(* Logix 5000 AddOnInstructionDefinition export Banner_IOLM_Param_C_v5; software revision 33.00 *)

TYPE Banner_IOL_Port_v5 :   // UDT that has all of the data items necessary to communicate with a specific Port on a IO-Link Master
STRUCT
   Port_Controlled : INT;   // Each bit represents a port on an IO-Link Master. Set to 1 to tell AOI to control that port.
   Port_Activate : INT;   // Each bit represents a port on an IO-Link Master. When ON that port will process any commands in queue.
   Port_Read : INT;   // Each bit represents a port on an IO-Link Master. Used to determine when device AOI has requested a Read command.
   Port_Write : INT;   // Each bit represents a port on an IO-Link Master. Used to determine when device AOI has requested a Write command.
   Port_RW_Complete : INT;   // Each bit represents a port on an IO-Link Master. Tells device AOI that Read or Write request has been completed.
   Port_Device_Read : INT;
   Data_Transfer : SINT[250];   // Array to transfer data from IO-Master to device AOIs.
END_STRUCT
END_TYPE

TYPE Banner_IOLM_EL_v5 :   // Error Log for Messages to IOLM.
STRUCT
   RW : SINT;   // 0 = Read, 1 = Write.
   Port : SINT;   // Port number that generated error.
   Index : INT;   // IO-Link Index for generated error.
END_STRUCT
END_TYPE

TYPE Banner_IOLMC_v5 :   // UDT to control IO-Link Masters. Modified for Comtrol Masters.
STRUCT
   Message_Source_Data : SINT[520];   // Array used to generate the source data for an Explicit Message
   Message_Destination_Data : SINT[520];   // Array that stores the data from the IO-Link sensor for an Explicit Message.
   Error_Log : Banner_IOLM_EL_v5[10];
   Error_Write_Retry : BOOL;
   Num_Error_MSGS : DINT;   // 0 = While waiting for a command, 1 = Processing command
   IO_Link_Master_Busy : BOOL;
   AOI_Reset : BOOL;   // Resets AOI.
   Port_Data : Banner_IOL_Port_v5;
   Halt_Operation : BOOL;
   AOI_Halted : BOOL;
END_STRUCT
END_TYPE

ADD_ON_INSTRUCTION Banner_IOLM_Param_C_v5   (* revision 5.0, vendor Banner Engineering *)
// AOI that controls a Comtrol IO-Link Master with Banner devices for parameter data operations.
VAR_IN_OUT
   Message : MESSAGE; {required}   // Message used to gather data from a device plugged into an Allen Bradley IO-Link Master.
   IOLM : Banner_IOLMC_v5; {required}
END_VAR
VAR_INPUT
   Port1 : BOOL; {required}
   Port2 : BOOL; {required}
   Port3 : BOOL; {required}
   Port4 : BOOL; {required}
   Port5 : BOOL; {required}
   Port6 : BOOL; {required}
   Port7 : BOOL; {required}
   Port8 : BOOL; {required}
END_VAR
VAR_OUTPUT
   Done : BOOL; {visible}
   Busy : BOOL; {visible}
   Error : BOOL; {visible}
END_VAR
VAR
   Lock : DINT; {access None}
   Disable_Timer : BOOL; {access None}
   Byte_Length : SINT; {access None}
   Current_Port : INT; {access None}   // Current port to communicate with via the IO-Link Master.
   Array_Index : DINT; {access None}
   Data_Index : DINT; {access None}
   Message_Timer : TIMER := (PRE := 100); {access None}
   Message_Timer2 : TIMER := (PRE := 5000); {access None}
   Error_Index : DINT; {access None}
   Temp_Index : INT; {access None}
   Timer8 : TIMER := (PRE := 3000); {access None}
   WriteCnt : DINT; {access None}
   Last_Index : DINT; {access None}
   WrCntTotal : DINT; {access None}
END_VAR

ROUTINE Logic   (* ladder *)
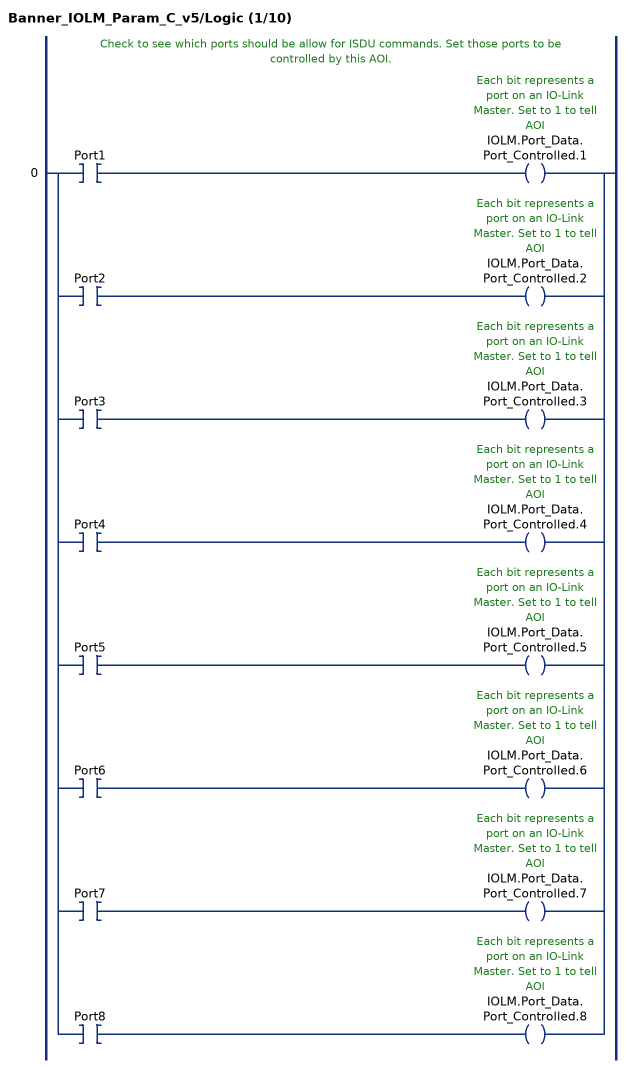
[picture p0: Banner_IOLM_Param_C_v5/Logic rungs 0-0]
   // Check to see which ports should be allow for ISDU commands. Set those ports to be controlled by this AOI.
   0: [XIC(Port1) OTE(IOLM.Port_Data.Port_Controlled.1) ,XIC(Port2) OTE(IOLM.Port_Data.Port_Controlled.2) ,XIC(Port3) OTE(IOLM.Port_Data.Port_Controlled.3) ,XIC(Port4) OTE(IOLM.Port_Data.Port_Controlled.4) ,XIC(Port5) OTE(IOLM.Port_Data.Port_Controlled.5) ,XIC(Port6) OTE(IOLM.Port_Data.Port_Controlled.6) ,XIC(Port7) OTE(IOLM.Port_Data.Port_Controlled.7) ,XIC(Port8) OTE(IOLM.Port_Data.Port_Controlled.8) ];
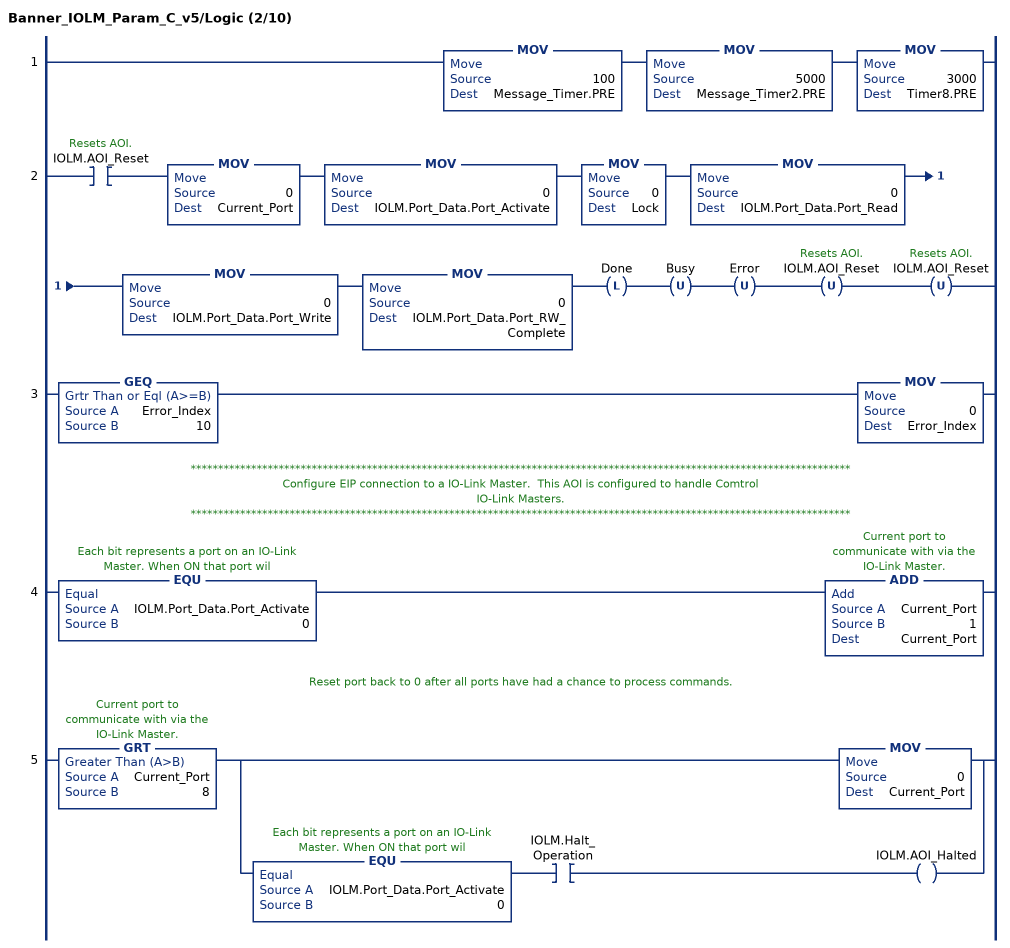
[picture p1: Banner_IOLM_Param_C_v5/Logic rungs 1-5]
   1: MOV(100,Message_Timer.PRE)MOV(5000,Message_Timer2.PRE)MOV(3000,Timer8.PRE);
   2: XIC(IOLM.AOI_Reset)MOV(0,Current_Port)MOV(0,IOLM.Port_Data.Port_Activate)MOV(0,Lock)MOV(0,IOLM.Port_Data.Port_Read)MOV(0,IOLM.Port_Data.Port_Write)MOV(0,IOLM.Port_Data.Port_RW_Complete)OTL(Done)OTU(Busy)OTU(Error)OTU(IOLM.AOI_Reset)OTU(IOLM.AOI_Reset);
   3: GEQ(Error_Index,10)MOV(0,Error_Index);
   // ************************************************************************************************************************
   // Configure EIP connection to a IO-Link Master.  This AOI is configured to handle Comtrol
   // IO-Link Masters.
   // ************************************************************************************************************************
   4: EQU(IOLM.Port_Data.Port_Activate,0)ADD(Current_Port,1,Current_Port);
   // Reset port back to 0 after all ports have had a chance to process commands.
   5: GRT(Current_Port,8)[MOV(0,Current_Port) ,EQU(IOLM.Port_Data.Port_Activate,0) XIC(IOLM.Halt_Operation) OTE(IOLM.AOI_Halted) ];
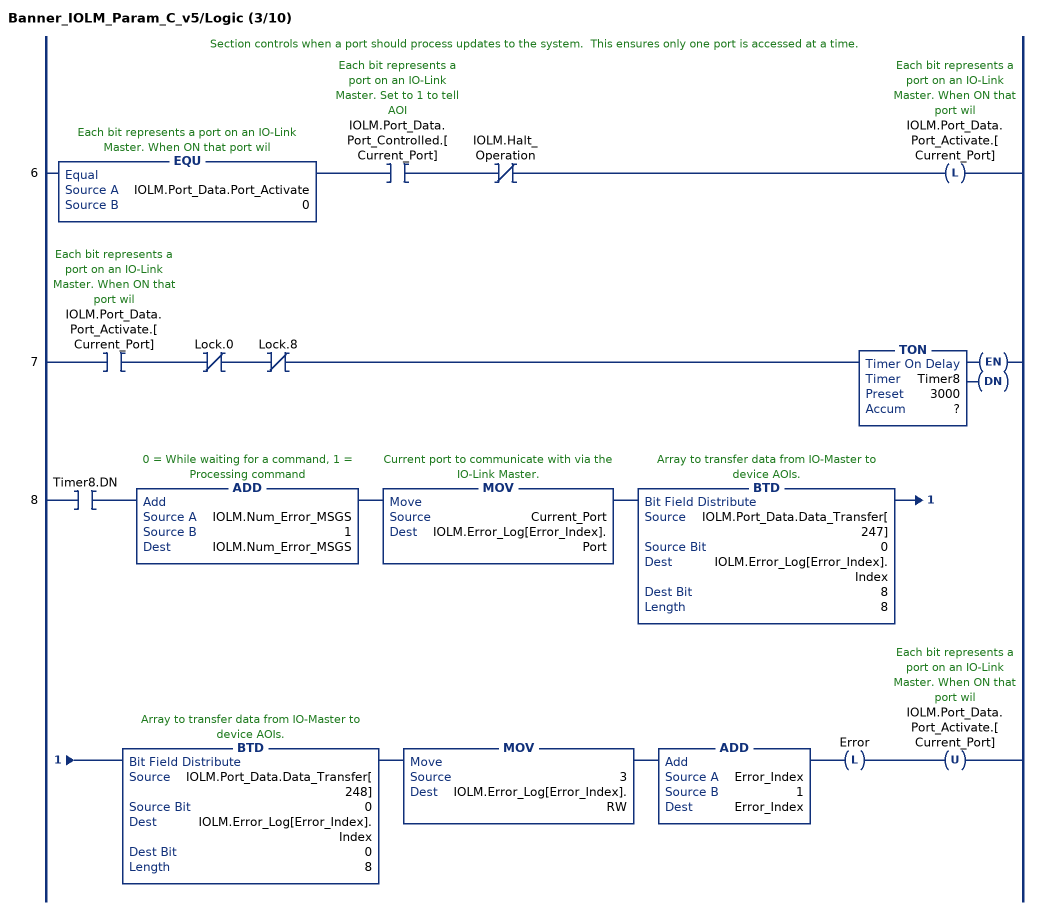
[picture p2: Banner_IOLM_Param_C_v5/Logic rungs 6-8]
   // Section controls when a port should process updates to the system.  This ensures only one port is accessed at a time.
   6: EQU(IOLM.Port_Data.Port_Activate,0)XIC(IOLM.Port_Data.Port_Controlled.[Current_Port])XIO(IOLM.Halt_Operation)OTL(IOLM.Port_Data.Port_Activate.[Current_Port]);
   7: XIC(IOLM.Port_Data.Port_Activate.[Current_Port])XIO(Lock.0)XIO(Lock.8)TON(Timer8,?,?);
   8: XIC(Timer8.DN)ADD(IOLM.Num_Error_MSGS,1,IOLM.Num_Error_MSGS)MOV(Current_Port,IOLM.Error_Log[Error_Index].Port)BTD(IOLM.Port_Data.Data_Transfer[247],0,IOLM.Error_Log[Error_Index].Index,8,8)BTD(IOLM.Port_Data.Data_Transfer[248],0,IOLM.Error_Log[Error_Index].Index,0,8)MOV(3,IOLM.Error_Log[Error_Index].RW)ADD(Error_Index,1,Error_Index)OTL(Error)OTU(IOLM.Port_Data.Port_Activate.[Current_Port]);
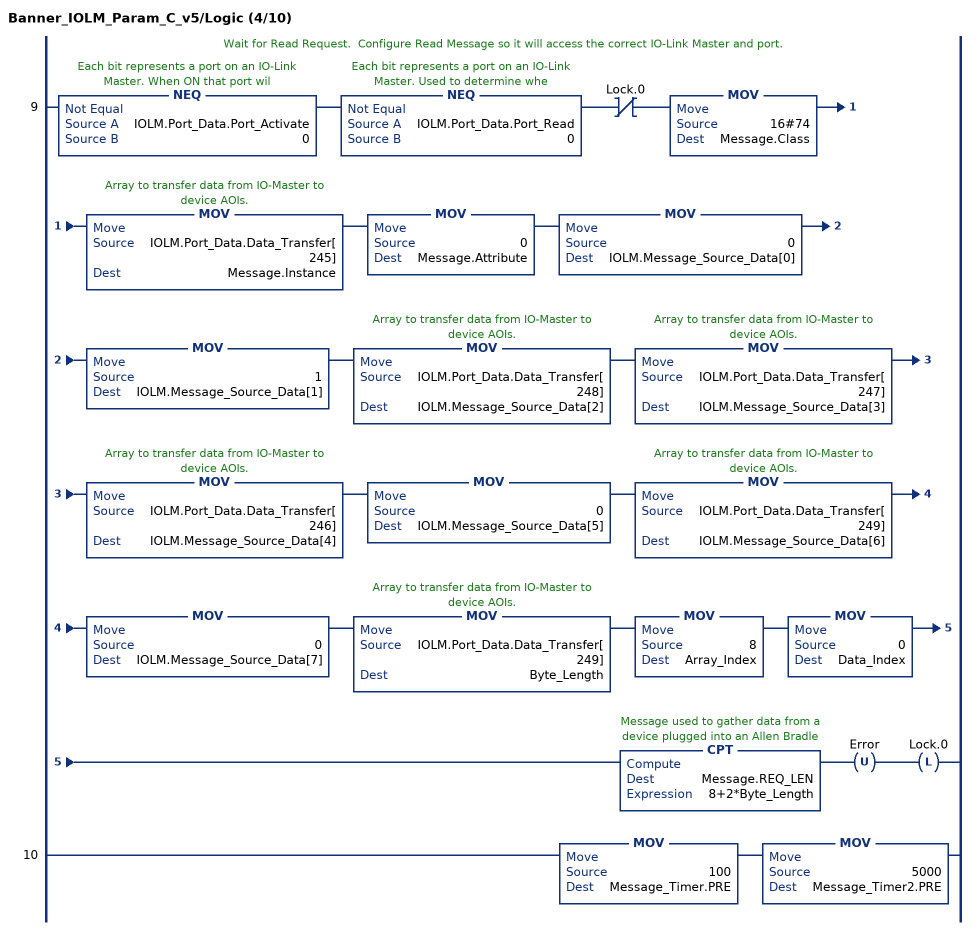
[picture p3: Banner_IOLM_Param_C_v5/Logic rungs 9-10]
   // Wait for Read Request.  Configure Read Message so it will access the correct IO-Link Master and port.
   9: NEQ(IOLM.Port_Data.Port_Activate,0)NEQ(IOLM.Port_Data.Port_Read,0)XIO(Lock.0)MOV(16#74,Message.Class)MOV(IOLM.Port_Data.Data_Transfer[245],Message.Instance)MOV(0,Message.Attribute)MOV(0,IOLM.Message_Source_Data[0])MOV(1,IOLM.Message_Source_Data[1])MOV(IOLM.Port_Data.Data_Transfer[248],IOLM.Message_Source_Data[2])MOV(IOLM.Port_Data.Data_Transfer[247],IOLM.Message_Source_Data[3])MOV(IOLM.Port_Data.Data_Transfer[246],IOLM.Message_Source_Data[4])MOV(0,IOLM.Message_Source_Data[5])MOV(IOLM.Port_Data.Data_Transfer[249],IOLM.Message_Source_Data[6])MOV(0,IOLM.Message_Source_Data[7])MOV(IOLM.Port_Data.Data_Transfer[249],Byte_Length)MOV(8,Array_Index)MOV(0,Data_Index)CPT(Message.REQ_LEN,8+2*Byte_Length)OTU(Error)OTL(Lock.0);
   10: MOV(100,Message_Timer.PRE)MOV(5000,Message_Timer2.PRE);
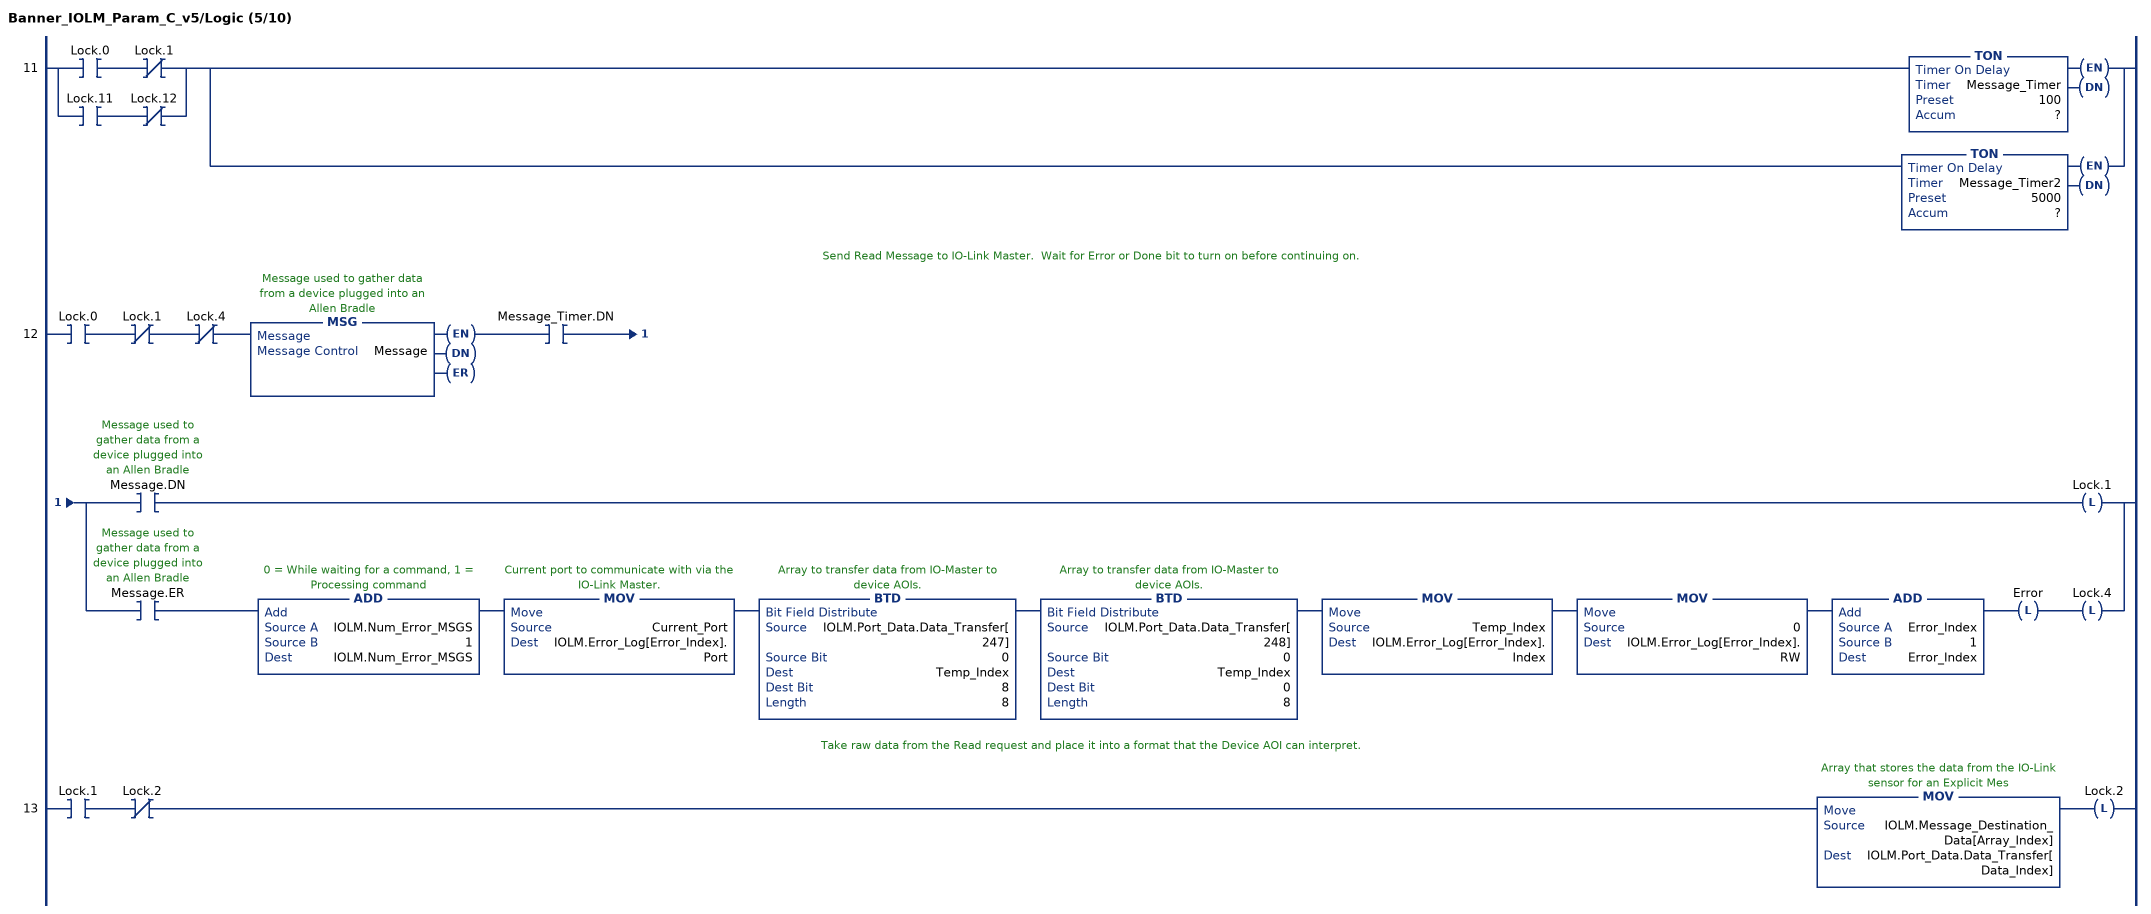
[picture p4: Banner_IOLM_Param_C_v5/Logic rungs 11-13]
   11: [XIC(Lock.0) XIO(Lock.1) ,XIC(Lock.11) XIO(Lock.12) ][TON(Message_Timer,?,?) ,TON(Message_Timer2,?,?) ];
   // Send Read Message to IO-Link Master.  Wait for Error or Done bit to turn on before continuing on.
   12: XIC(Lock.0)XIO(Lock.1)XIO(Lock.4)MSG(Message)XIC(Message_Timer.DN)[XIC(Message.DN) OTL(Lock.1) ,XIC(Message.ER) ADD(IOLM.Num_Error_MSGS,1,IOLM.Num_Error_MSGS) MOV(Current_Port,IOLM.Error_Log[Error_Index].Port) BTD(IOLM.Port_Data.Data_Transfer[247],0,Temp_Index,8,8) BTD(IOLM.Port_Data.Data_Transfer[248],0,Temp_Index,0,8) MOV(Temp_Index,IOLM.Error_Log[Error_Index].Index) MOV(0,IOLM.Error_Log[Error_Index].RW) ADD(Error_Index,1,Error_Index) OTL(Error) OTL(Lock.4) ];
   // Take raw data from the Read request and place it into a format that the Device AOI can interpret.
   13: XIC(Lock.1)XIO(Lock.2)MOV(IOLM.Message_Destination_Data[Array_Index],IOLM.Port_Data.Data_Transfer[Data_Index])OTL(Lock.2);
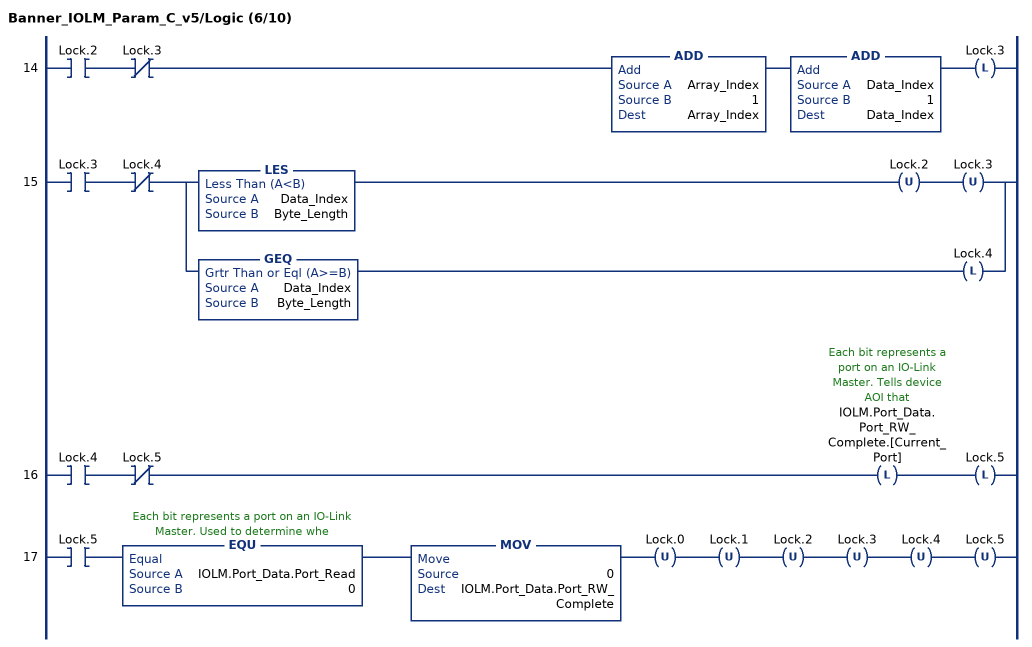
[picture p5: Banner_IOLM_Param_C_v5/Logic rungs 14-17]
   14: XIC(Lock.2)XIO(Lock.3)ADD(Array_Index,1,Array_Index)ADD(Data_Index,1,Data_Index)OTL(Lock.3);
   15: XIC(Lock.3)XIO(Lock.4)[LES(Data_Index,Byte_Length) OTU(Lock.2) OTU(Lock.3) ,GEQ(Data_Index,Byte_Length) OTL(Lock.4) ];
   16: XIC(Lock.4)XIO(Lock.5)OTL(IOLM.Port_Data.Port_RW_Complete.[Current_Port])OTL(Lock.5);
   17: XIC(Lock.5)EQU(IOLM.Port_Data.Port_Read,0)MOV(0,IOLM.Port_Data.Port_RW_Complete)OTU(Lock.0)OTU(Lock.1)OTU(Lock.2)OTU(Lock.3)OTU(Lock.4)OTU(Lock.5);
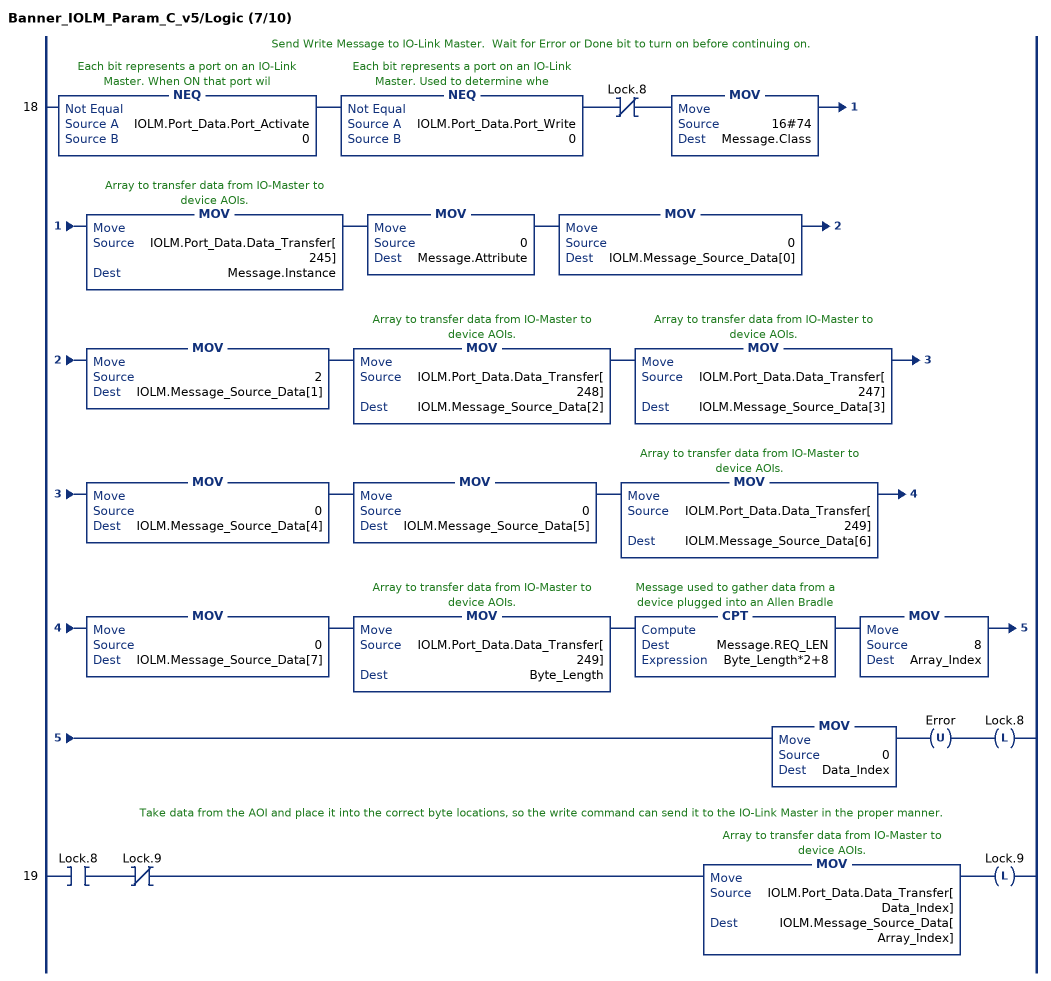
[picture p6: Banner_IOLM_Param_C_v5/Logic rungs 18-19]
   // Send Write Message to IO-Link Master.  Wait for Error or Done bit to turn on before continuing on.
   18: NEQ(IOLM.Port_Data.Port_Activate,0)NEQ(IOLM.Port_Data.Port_Write,0)XIO(Lock.8)MOV(16#74,Message.Class)MOV(IOLM.Port_Data.Data_Transfer[245],Message.Instance)MOV(0,Message.Attribute)MOV(0,IOLM.Message_Source_Data[0])MOV(2,IOLM.Message_Source_Data[1])MOV(IOLM.Port_Data.Data_Transfer[248],IOLM.Message_Source_Data[2])MOV(IOLM.Port_Data.Data_Transfer[247],IOLM.Message_Source_Data[3])MOV(0,IOLM.Message_Source_Data[4])MOV(0,IOLM.Message_Source_Data[5])MOV(IOLM.Port_Data.Data_Transfer[249],IOLM.Message_Source_Data[6])MOV(0,IOLM.Message_Source_Data[7])MOV(IOLM.Port_Data.Data_Transfer[249],Byte_Length)CPT(Message.REQ_LEN,Byte_Length*2+8)MOV(8,Array_Index)MOV(0,Data_Index)OTU(Error)OTL(Lock.8);
   // Take data from the AOI and place it into the correct byte locations, so the write command can send it to the IO-Link Master in the proper manner.
   19: XIC(Lock.8)XIO(Lock.9)MOV(IOLM.Port_Data.Data_Transfer[Data_Index],IOLM.Message_Source_Data[Array_Index])OTL(Lock.9);
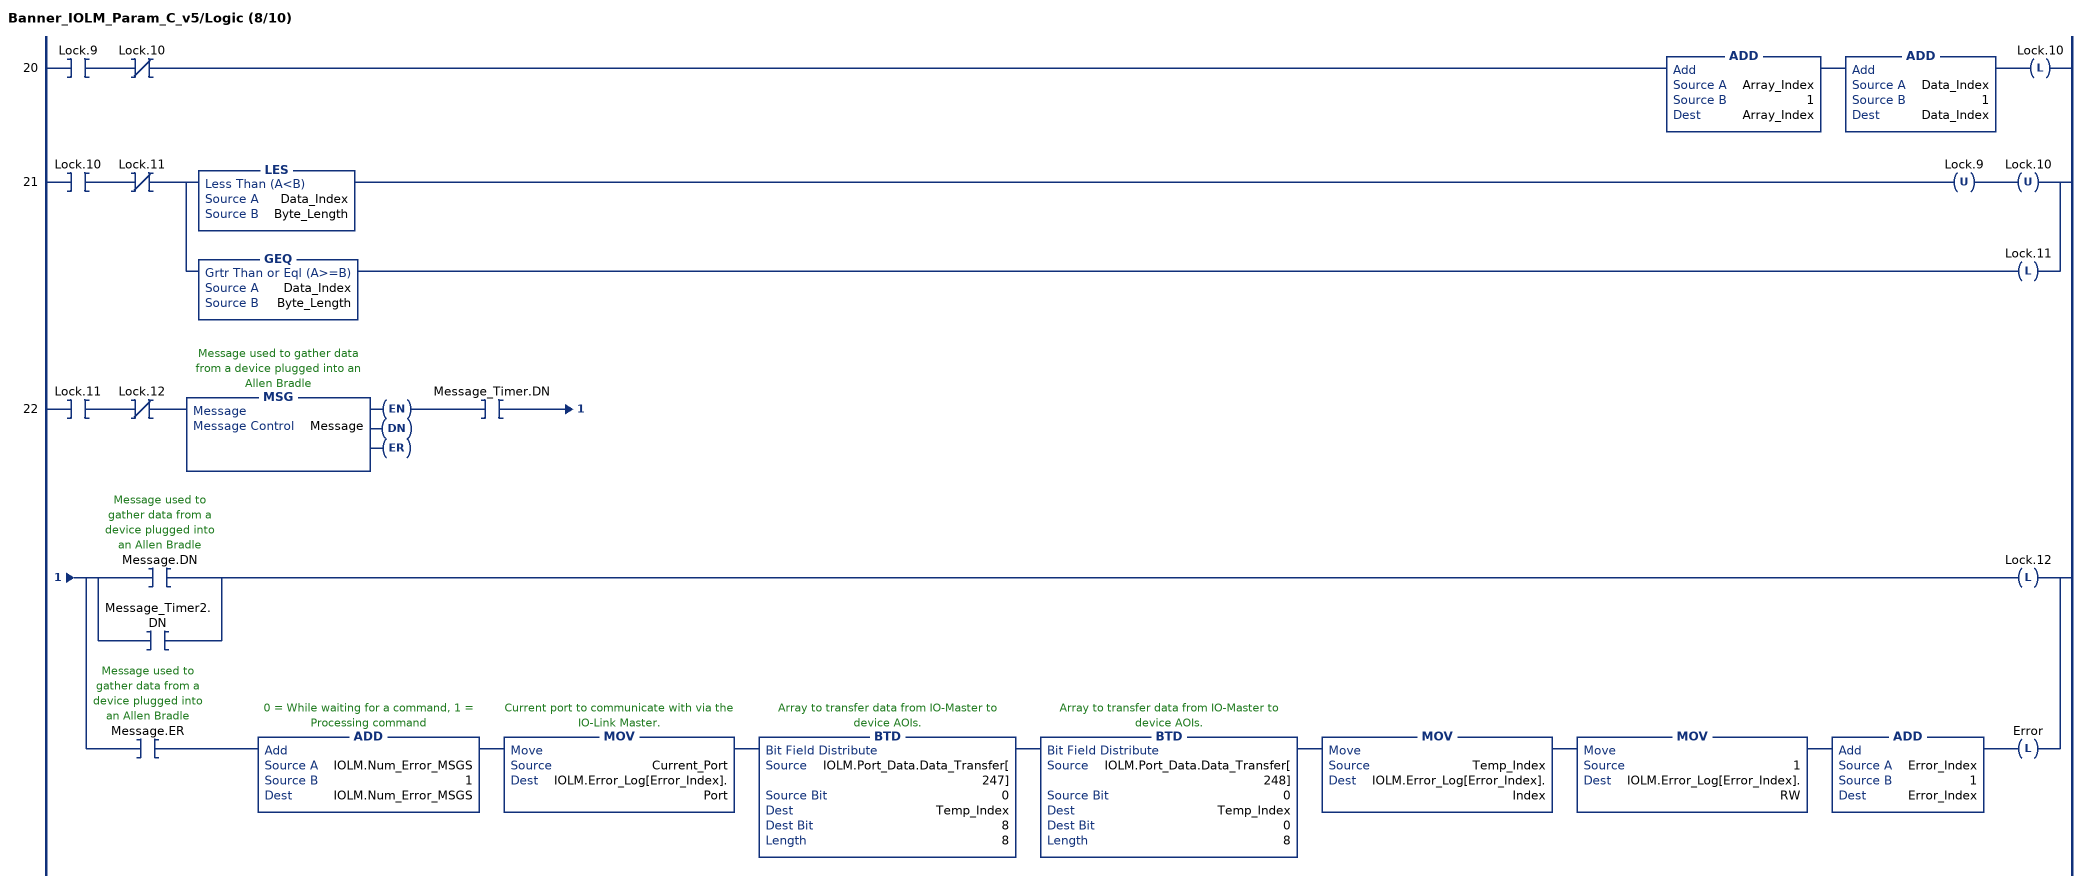
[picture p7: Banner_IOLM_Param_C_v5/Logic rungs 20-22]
   20: XIC(Lock.9)XIO(Lock.10)ADD(Array_Index,1,Array_Index)ADD(Data_Index,1,Data_Index)OTL(Lock.10);
   21: XIC(Lock.10)XIO(Lock.11)[LES(Data_Index,Byte_Length) OTU(Lock.9) OTU(Lock.10) ,GEQ(Data_Index,Byte_Length) OTL(Lock.11) ];
   22: XIC(Lock.11)XIO(Lock.12)MSG(Message)XIC(Message_Timer.DN)[[XIC(Message.DN) ,XIC(Message_Timer2.DN) ] OTL(Lock.12) ,XIC(Message.ER) ADD(IOLM.Num_Error_MSGS,1,IOLM.Num_Error_MSGS) MOV(Current_Port,IOLM.Error_Log[Error_Index].Port) BTD(IOLM.Port_Data.Data_Transfer[247],0,Temp_Index,8,8) BTD(IOLM.Port_Data.Data_Transfer[248],0,Temp_Index,0,8) MOV(Temp_Index,IOLM.Error_Log[Error_Index].Index) MOV(1,IOLM.Error_Log[Error_Index].RW) ADD(Error_Index,1,Error_Index) OTL(Error) ];
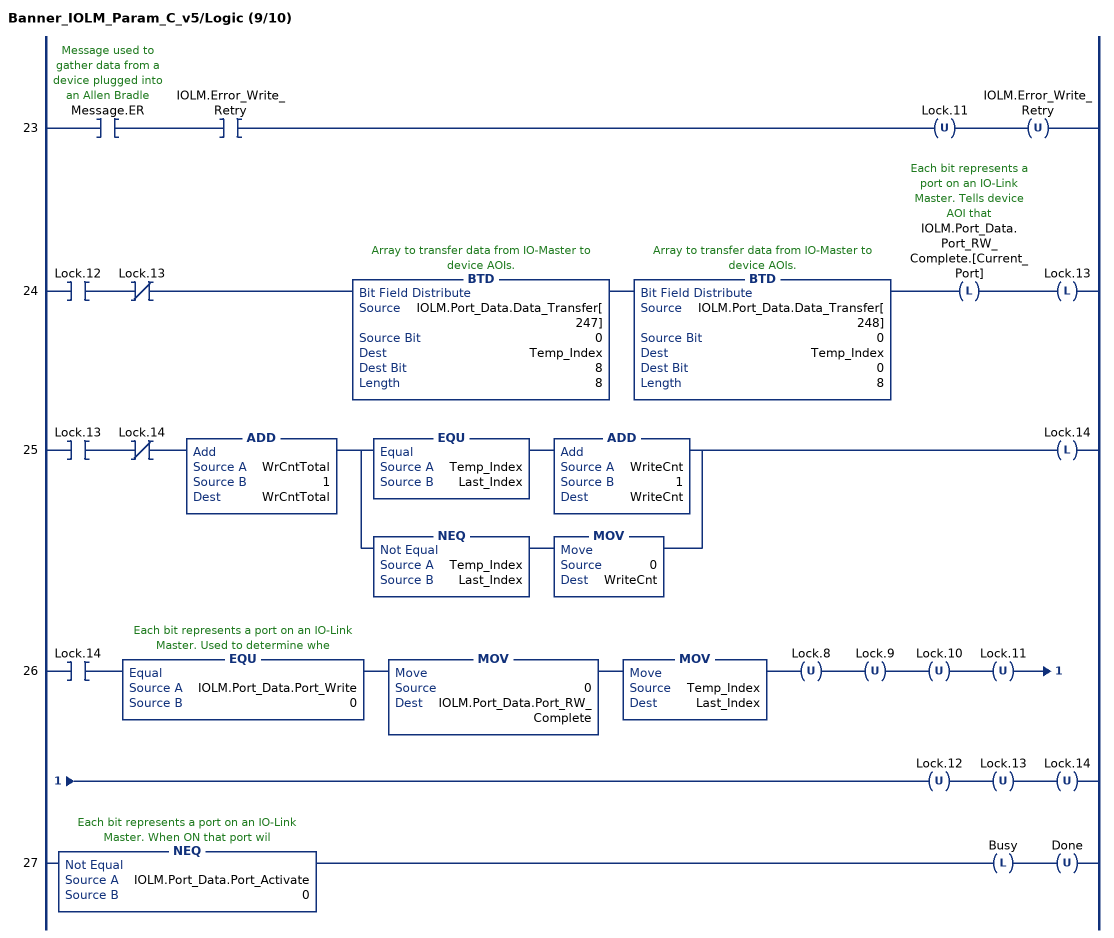
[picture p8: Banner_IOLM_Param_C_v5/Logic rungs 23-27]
   23: XIC(Message.ER)XIC(IOLM.Error_Write_Retry)OTU(Lock.11)OTU(IOLM.Error_Write_Retry);
   24: XIC(Lock.12)XIO(Lock.13)BTD(IOLM.Port_Data.Data_Transfer[247],0,Temp_Index,8,8)BTD(IOLM.Port_Data.Data_Transfer[248],0,Temp_Index,0,8)OTL(IOLM.Port_Data.Port_RW_Complete.[Current_Port])OTL(Lock.13);
   25: XIC(Lock.13)XIO(Lock.14)ADD(WrCntTotal,1,WrCntTotal)[EQU(Temp_Index,Last_Index) ADD(WriteCnt,1,WriteCnt) ,NEQ(Temp_Index,Last_Index) MOV(0,WriteCnt) ]OTL(Lock.14);
   26: XIC(Lock.14)EQU(IOLM.Port_Data.Port_Write,0)MOV(0,IOLM.Port_Data.Port_RW_Complete)MOV(Temp_Index,Last_Index)OTU(Lock.8)OTU(Lock.9)OTU(Lock.10)OTU(Lock.11)OTU(Lock.12)OTU(Lock.13)OTU(Lock.14);
   27: NEQ(IOLM.Port_Data.Port_Activate,0)OTL(Busy)OTU(Done);
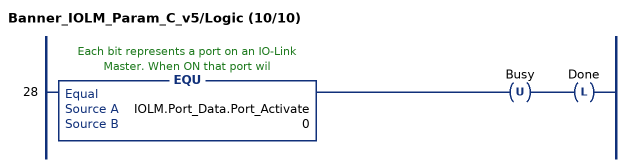
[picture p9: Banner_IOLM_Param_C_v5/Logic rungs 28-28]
   28: EQU(IOLM.Port_Data.Port_Activate,0)OTU(Busy)OTL(Done);
END_ROUTINE
END_ADD_ON_INSTRUCTION
